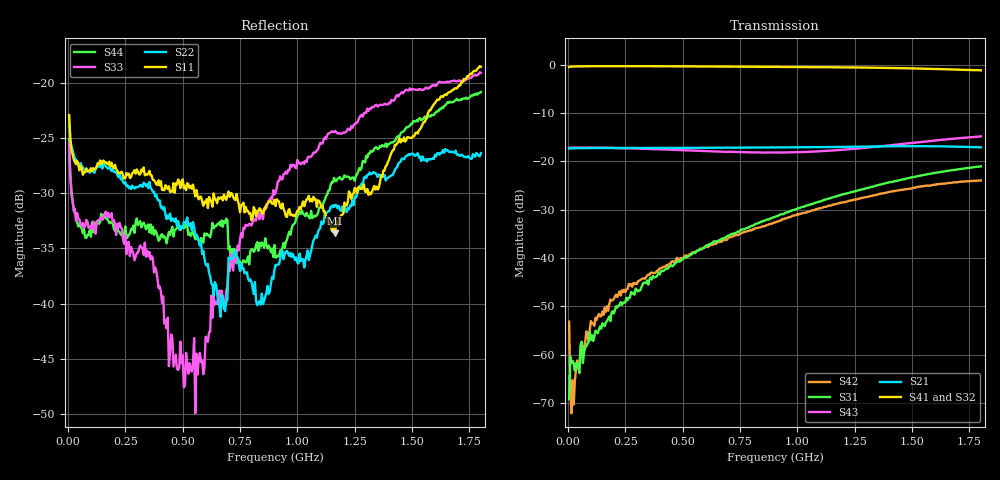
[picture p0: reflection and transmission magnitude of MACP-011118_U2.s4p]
!Agilent Technologies,E5071C,MY46110647,A.11.31
!Date: Thu Jan 18 12:37:10 2024 DD
!Data & Calibration Information:
!MACP-011118 soldered onto PT-0003645 with F connectors, Calibration PT-0003645-TRL. Port1 (pin3) Port2 (pin1) Port3 (pin6) Port4 (pin4)
!Freq	S11:SOLT4(ON)	S12:SOLT4(ON)	S13:SOLT4(ON)	S14:SOLT4(ON)
!	S21:SOLT4(ON)	S22:SOLT4(ON)	S23:SOLT4(ON)	S24:SOLT4(ON)
!	S31:SOLT4(ON)	S32:SOLT4(ON)	S33:SOLT4(ON)	S34:SOLT4(ON)
!	S41:SOLT4(ON)	S42:SOLT4(ON)	S43:SOLT4(ON)	S44:SOLT4(ON)
!PortZ  Port1:75+j0  Port2:75+j0  Port3:75+j0  Port4:75+j0
!Above PortZ is port z conversion or system Z0 setting when saving the data.
!When reading, reference impedance value at option line is always used.
# Hz S MA R 75
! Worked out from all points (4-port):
!   360 points, 5 MHz to 1.8 GHz, reference 75 ohm
!   strongest paths, dB at 5 MHz, 455 MHz, 905 MHz, 1.355 GHz, 1.8 GHz:
!     S41: -0.5, -0.3, -0.5, -0.7, -1.2
!     S32: -0.5, -0.4, -0.5, -0.8, -1.4
!     S21: -17.3, -17.2, -17.1, -16.9, -17.1
!     S43: -17.2, -17.6, -18.2, -16.9, -14.8
!     S31: -69.2, -41.7, -31.4, -24.9, -21.0
!     S42: -53.2, -40.6, -32.6, -26.8, -24.0
!   lowest |S11| = -33.6 dB at 1.165 GHz (marker M1), VSWR 1.04, Z = 72.2 + j1.21 ohm
!   |S11| at or under -10 dB: start of sweep to end of sweep
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5000000  0.07143 146.2  0.1334 -177.8  0.001813 -120.2  0.9457 2.3
         0.1358 -177.7  0.07115 148.1  0.9475 2.2  0.001177 -63.3
         0.0003466 61.3  0.9446 2.2  0.05332 132.2  0.1384 2.0
         0.9451 2.3  0.002199 -70.5  0.1387 1.9  0.05555 135.9
1.5e7  0.04997 161.0  0.1361 -179.8  0.0005894 -140.3  0.9546 0.7
       0.1362 -179.9  0.05168 160.8  0.9546 0.7  0.0004471 -137.4
       0.0008158 -117.8  0.9549 0.7  0.03101 150.5  0.1384 0.6
       0.9549 0.7  0.0002479 -128.5  0.1385 0.6  0.03289 150.4
1e8  0.04103 163.6  0.1373 172.8  0.001082 127.0  0.9626 -2.5
     0.1374 172.8  0.03987 171.9  0.9626 -2.6  0.001936 117.4
     0.001424 146.3  0.9627 -2.6  0.02251 169.8  0.1385 -1.2
     0.9628 -2.5  0.002233 109.0  0.1385 -1.1  0.02008 154.8
5.55e8  0.03061 129.6  0.1379 138.8  0.01128 113.8  0.9596 -15.9
        0.1379 138.8  0.02055 176.8  0.9555 -16.4  0.01117 87.7
        0.01124 117.8  0.9565 -16.4  0.003186 -139.5  0.129 -4.7
        0.9596 -15.9  0.01143 87.2  0.1289 -4.8  0.01958 73.5
7.65e8  0.02866 139.8  0.1387 123.5  0.01945 100.7  0.9542 -22.1
        0.1385 123.3  0.01448 -151.2  0.9491 -22.5  0.01753 76.5
        0.01997 105.7  0.9499 -22.5  0.02206 -78.6  0.1244 -3.5
        0.9547 -22.1  0.01846 73.1  0.1243 -3.5  0.01571 45.8
1.165e9  0.02083 156.3  0.1409 94.2  0.0419 78.2  0.9393 -33.8
         0.141 94.1  0.02802 -81.6  0.9234 -34.7  0.03334 52.9
         0.04314 81.1  0.9248 -34.7  0.0606 -92.0  0.1298 3.2
         0.9388 -33.8  0.03606 52.6  0.1302 3.0  0.03585 -41.8
1.8e9  0.1182 174.9  0.14 41.8  0.08758 28.5  0.8745 -53.7
       0.1396 41.5  0.04806 -108.9  0.8518 -53.6  0.05956 0.6
       0.08868 29.2  0.853 -53.9  0.111 -135.2  0.1804 -2.8
       0.8739 -53.8  0.06344 1.8  0.1812 -2.8  0.09081 -102.4
